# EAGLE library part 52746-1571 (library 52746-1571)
Molex FFC/FPC SMT Series 0.5mm Pitch 15 Way 1 Row Right Angle SMT Female PCB Housing, Gold over Nickel Plated Contacts Source: Datasheet
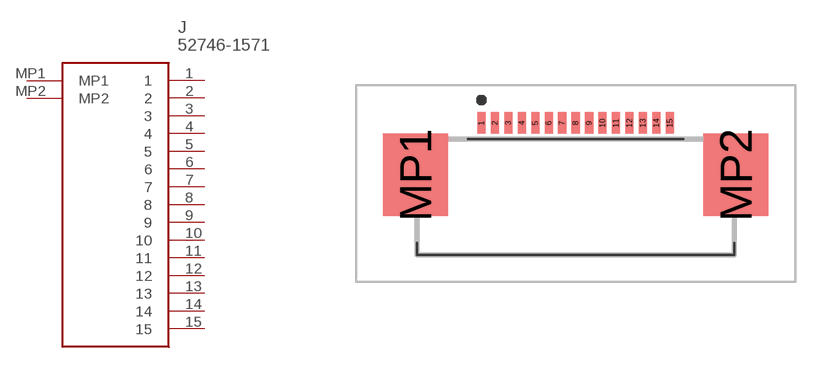
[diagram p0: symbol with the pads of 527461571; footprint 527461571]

Designator prefix J

## 52746-1571 (Description: Molex FFC/FPC SMT Series 0.5mm Pitch 15 Way 1 Row Right Angle SMT Female PCB Housing, Gold over Nickel Plated Contacts; Height: 2.2mm; Manufacturer_Name: Molex; Manufacturer_Part_Number: 52746-1571; Mouser_Part_Number: 538-52746-1571; Mouser_Price-Stock: https://www.mouser.co.uk/ProductDetail/Molex/52746-1571?qs=nDwhpid8gJZ2Rlv1mA0S1w%3D%3D)  [527461571]
1  1
2  2
3  3
4  4
5  5
6  6
7  7
8  8
9  9
10  10
11  11
12  12
13  13
14  14
15  15
MP1  MP1
MP2  MP2

## Footprint 527461571 (pad centres in mm)
52746-1571-1
smd 0.3 x 0.8: 1 -3.5,2.45; 2 -3,2.45; 3 -2.5,2.45; 4 -2,2.45; 5 -1.5,2.45; 6 -1,2.45; 7 -0.5,2.45; 8 0,2.45; 9 0.5,2.45; 10 1,2.45; 11 1.5,2.45; 12 2,2.45; 13 2.5,2.45; 14 3,2.45; 15 3.5,2.45
smd 2.4 x 3.05: MP1 -5.95,0.525; MP2 5.95,0.525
